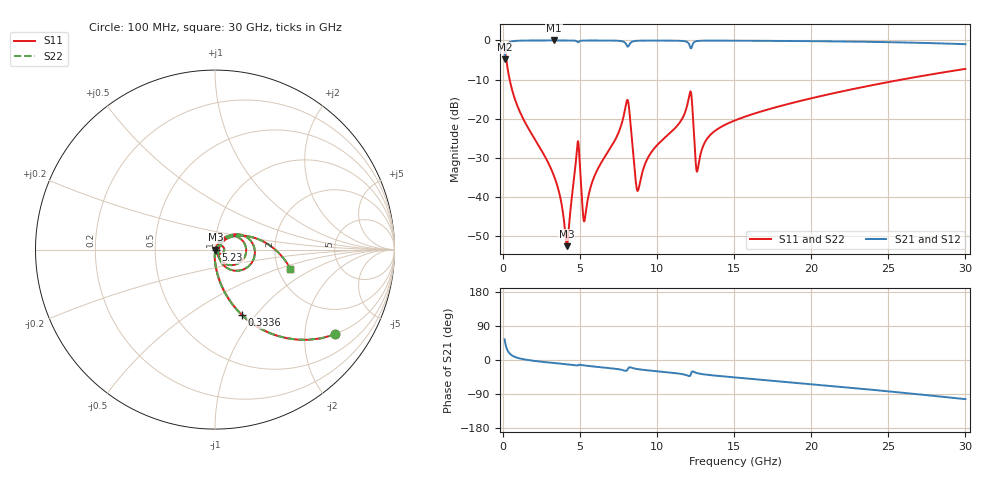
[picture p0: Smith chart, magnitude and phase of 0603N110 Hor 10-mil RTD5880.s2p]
# GHz S MA R 50
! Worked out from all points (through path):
!   3201 points, 100 MHz to 30 GHz, reference 50 ohm
!   highest |S21| = -0.02 dB at 3.305 GHz (marker M1); lowest = -4.9 dB at 100 MHz (marker M2)
!   group delay of S21, straight-line fit = 9.97 ps
!   lowest |S11| = -52.5 dB at 4.146 GHz (marker M3), VSWR 1.00, Z = 50.2 - j0.0561 ohm
!   |S11| at or under -10 dB: 426.2 MHz to 25.85 GHz (25.43 GHz wide, 194 % of centre)
!   |S22| runs from -52.5 to -1.7 dB; largest |S21 - S12| = 0
!   S11 on the Smith chart (normalised r, x): 100 MHz: 0.99, -2.85; 333.6 MHz: 0.99, -0.85; 5.23 GHz: 1.01, -0.00; 30 GHz: 2.34, -0.61
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0.1  0.82 -35.2  0.5721 54.8  0.5721 54.8  0.82 -35.2
0.3335938  0.393 -67.7  0.9191 22.2  0.9191 22.2  0.393 -67.7
1.07175  0.1253 -85.3  0.9912 4.3  0.9912 4.3  0.1253 -85.3
3.304906  0.01869 -92.7  0.998 -8.0  0.998 -8.0  0.01869 -92.7
4.145844  0.002379 -13.6  0.9976 -11.3  0.9976 -11.3  0.002379 -13.6
4.799906  0.04262 30.2  0.9693 -14.9  0.9693 -14.9  0.04262 30.2
4.930719  0.03877 -37.9  0.9647 -12.5  0.9647 -12.5  0.03877 -37.9
5.089563  0.01175 -54.0  0.991 -13.5  0.991 -13.5  0.01175 -54.0
5.229719  0.005109 -13.3  0.9948 -14.3  0.9948 -14.3  0.005109 -13.3
8.0235  0.1676 12.1  0.8659 -28.1  0.8659 -28.1  0.1676 12.1
8.191688  0.1276 -42.7  0.8813 -19.4  0.8813 -19.4  0.1276 -42.7
8.733625  0.01203 -3.6  0.9886 -24.0  0.9886 -24.0  0.01203 -3.6
10.06978  0.0478 54.4  0.9941 -30.1  0.9941 -30.1  0.0478 54.4
11.49938  0.09177 48.3  0.9873 -36.4  0.9873 -36.4  0.09177 48.3
12.10672  0.2093 11.2  0.8615 -42.5  0.8615 -42.5  0.2093 11.2
12.24687  0.1764 -41.9  0.826 -31.3  0.826 -31.3  0.1764 -41.9
12.62063  0.02217 6.6  0.9831 -35.0  0.9831 -35.0  0.02217 6.6
13.34944  0.05942 45.1  0.9924 -39.4  0.9924 -39.4  0.05942 45.1
15.05  0.09551 41.5  0.991 -46.0  0.991 -46.0  0.09551 41.5
20.03956  0.1835 24.6  0.978 -63.9  0.978 -63.9  0.1835 24.6
25.01978  0.2948 6.1  0.9495 -82.8  0.9495 -82.8  0.2948 6.1
30  0.433 -14.2  0.8942 -103.3  0.8942 -103.3  0.433 -14.2
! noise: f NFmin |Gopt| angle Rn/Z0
0.1  0.000319  0.9252  0.523  0.0009458
3.417  0.003646  0.7917  9.381  0.003587
6.743  0.007456  0.799  18.35  0.007491
10.06  0.01002  0.7806  27.24  0.008853
13.39  0.01263  0.7716  36.02  0.01022
16.7  0.01251  0.723  44.4  0.007714
20.03  0.01445  0.7167  52.66  0.00815
23.35  0.01662  0.7165  60.69  0.008706
26.67  0.019  0.7198  68.53  0.009282
30  0.02163  0.7259  76.15  0.009867
